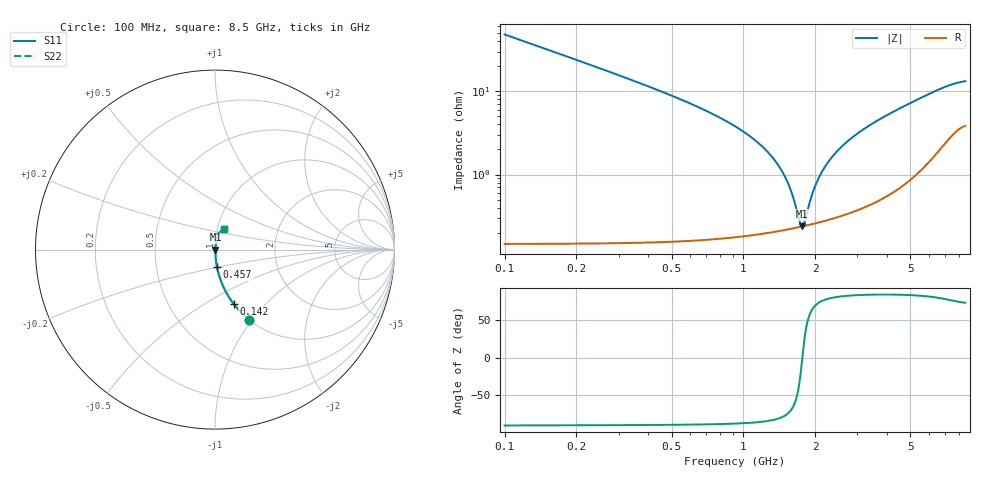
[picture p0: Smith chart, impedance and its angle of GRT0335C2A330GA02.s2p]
!Murata Part Number: GRT0335C2A330GA02
!These Parameters are Measured in Series Mode Connection
!Data Generated on Jun 19, 2026
!  o--ll--o
!Port1  Port2
!  o------o
!Operation Temp=25[degC], DC Bias Voltage=0[V]
!Freq. Start=100[MHz] Stop=9[GHz] 401[Steps]
# Hz S RI R 50
!Freq.(Hz) S11(Real) S11(Imag) S21(Real) S21(Imag) S12(Real) S12(Imag) S22(Real) S22(Imag)
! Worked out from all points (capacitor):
!   401 points, 100 MHz to 8.5 GHz, reference 50 ohm
!   read as one part in series: C = 33 pF near 142 MHz
!   lowest |Z| = 238 mohm at 1.759 GHz (marker M1)
!   series resonance near 1.764 GHz, so ESL is about 250 pH
!   S11 on the Smith chart (normalised r, x): 100 MHz: 1.00, -0.96; 142 MHz: 1.00, -0.67; 457 MHz: 1.00, -0.20; 8.5 GHz: 1.08, +0.25
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1e8  0.1885 -0.3896  0.8115 0.3896  0.8115 0.3896  0.1885 -0.3896
1.42e8  0.1033 -0.3021  0.8967 0.3021  0.8967 0.3021  0.1033 -0.3021
1.84e8  0.0642 -0.2422  0.9358 0.2422  0.9358 0.2422  0.0642 -0.2422
2.68e8  0.0313 -0.17  0.9687 0.17  0.9687 0.17  0.0313 -0.17
4.57e8  0.0111 -0.0972  0.9889 0.0972  0.9889 0.0972  0.0111 -0.0972
1.213e9  0.00238 -0.0209  0.9976 0.0209  0.9976 0.0209  0.00238 -0.0209
1.381e9  0.00225 -0.0135  0.9978 0.0135  0.9978 0.0135  0.00225 -0.0135
1.507e9  0.00224 -0.00861  0.9978 0.00861  0.9978 0.00861  0.00224 -0.00861
1.591e9  0.00226 -0.00563  0.9977 0.00563  0.9977 0.00563  0.00226 -0.00563
1.717e9  0.00234 -0.00147  0.9977 0.00147  0.9977 0.00147  0.00234 -0.00147
1.759e9  0.00237 -0.000158  0.9976 0.000158  0.9976 0.000158  0.00237 -0.000158
1.801e9  0.00241 0.00113  0.9976 -0.00113  0.9976 -0.00113  0.00241 0.00113
1.906e9  0.00252 0.00422  0.9975 -0.00422  0.9975 -0.00422  0.00252 0.00422
1.99e9  0.00262 0.00658  0.9974 -0.00658  0.9974 -0.00658  0.00262 0.00658
2.179e9  0.00289 0.0116  0.9971 -0.0116  0.9971 -0.0116  0.00289 0.0116
2.494e9  0.00346 0.0193  0.9965 -0.0193  0.9965 -0.0193  0.00346 0.0193
2.914e9  0.00442 0.0287  0.9956 -0.0287  0.9956 -0.0287  0.00442 0.0287
3.502e9  0.00617 0.0409  0.9938 -0.0409  0.9938 -0.0409  0.00617 0.0409
4.3e9  0.00947 0.0567  0.9905 -0.0567  0.9905 -0.0567  0.00947 0.0567
5.707e9  0.0192 0.0834  0.9808 -0.0834  0.9808 -0.0834  0.0192 0.0834
7.114e9  0.0361 0.1057  0.9639 -0.1057  0.9639 -0.1057  0.0361 0.1057
8.5e9  0.051 0.1153  0.949 -0.1153  0.949 -0.1153  0.051 0.1153
